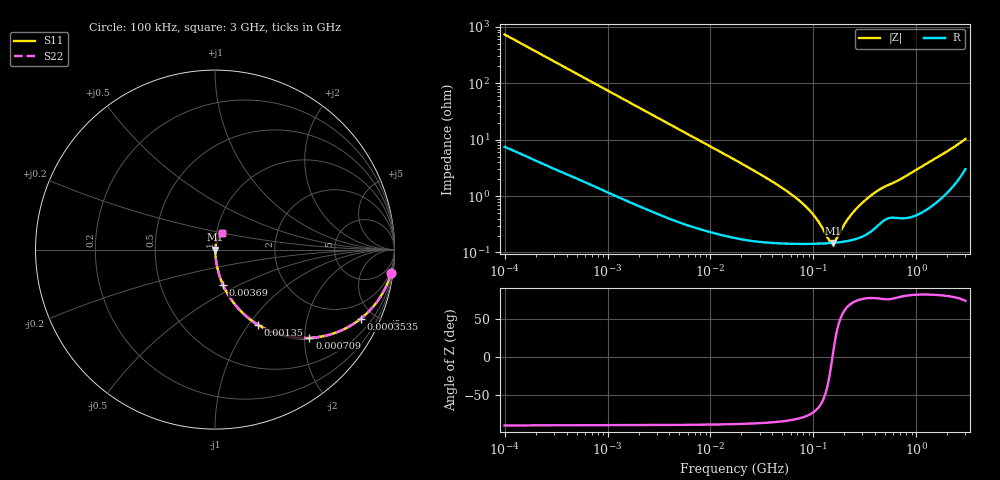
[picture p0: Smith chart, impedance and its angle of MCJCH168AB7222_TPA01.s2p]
! MCJCH168AB7222_TPA01  S-PARAMETER MODEL  ( Standard Model )
! Model Generated by TAIYO YUDEN Corporation (http://www.ty-top.com)
! Version 1.0
! TAIYO YUDEN Control No. 220601
! Copyright(c) 2015 TAIYO YUDEN CO.,LTD. All Rights Reserved.
! Product Description (link to TY-COMPAS)
! https://ds.yuden.co.jp/TYCOMPAS/or/detail?pn=MCJCH168AB7222KTPA01&u=M
! Products Name : Multilayer Ceramic Capacitors
! Characteristics :
!  Capacitance : 2200 [pF] , Rated Voltage : 100 [V] , TCC : X7R
!  Case Size : 1.6 x 0.8 / 0.063 x 0.031 [mm/inch] , Thickness : 0.8 / 0.031 [mm/inch]
!  (Conditions: Temperature = 25 [degC] , DC Bias Voltage = 0 [V])
! External Node Assignments :
!  1  o---| |---o  2
! GND o---------o GND
! Frequency Range : 100kHz  -  3GHz  [ 401 STEP ]
# MHZ S RI R 50
! Freq[MHz].  S11 Real  S11 Imag  S21 Real  S21 Imag  S12 Real  S12 Imag  S22 Real  S22 Imag
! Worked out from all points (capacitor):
!   401 points, 100 kHz to 3 GHz, reference 50 ohm
!   read as one part in series: C = 2.16 nF near 105.3 kHz
!   lowest |Z| = 148 mohm at 154.9 MHz (marker M1)
!   series resonance near 153.4 MHz, so ESL is about 500 pH
!   S11 on the Smith chart (normalised r, x): 100 kHz: 1, -15; 353.5 kHz: 1.05, -4.20; 709 kHz: 1.03, -2.11; 1.35 MHz: 1.02, -1.11; 3.69 MHz: 1.01, -0.41; 3 GHz: 1.06, +0.20
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0.1  0.9805 -0.1331  0.0195 0.1331  0.0195 0.1331  0.9805 -0.1331
0.205778  0.9256 -0.2568  0.0744 0.2568  0.0744 0.2568  0.9256 -0.2568
0.353547  0.812 -0.3844  0.188 0.3844  0.188 0.3844  0.812 -0.3844
0.562235  0.6354 -0.4743  0.3646 0.4743  0.3646 0.4743  0.6354 -0.4743
0.709011  0.5256 -0.492  0.4744 0.492  0.4744 0.492  0.5256 -0.492
1.350433  0.24 -0.4189  0.76 0.4189  0.76 0.4189  0.24 -0.4189
1.987766  0.1301 -0.3277  0.8699 0.3277  0.8699 0.3277  0.1301 -0.3277
3.161081  0.0582 -0.2245  0.9418 0.2245  0.9418 0.2245  0.0582 -0.2245
3.689712  0.0442 -0.1956  0.9558 0.1956  0.9558 0.1956  0.0442 -0.1956
7.399428  0.0131 -0.1013  0.9869 0.1013  0.9869 0.1013  0.0131 -0.1013
17.7727  0.00359 -0.0425  0.9964 0.0425  0.9964 0.0425  0.00359 -0.0425
53.83243  0.00159 -0.0126  0.9984 0.0126  0.9984 0.0126  0.00159 -0.0126
75.25761  0.00148 -0.00779  0.9985 0.00779  0.9985 0.00779  0.00148 -0.00779
97.38194  0.00144 -0.00474  0.9986 0.00474  0.9986 0.00474  0.00144 -0.00474
143.341  0.00146 -0.000687  0.9985 0.000687  0.9985 0.000687  0.00146 -0.000687
154.8634  0.00148 9.42e-05  0.9985 -9.42e-05  0.9985 -9.42e-05  0.00148 9.42e-05
167.3121  0.0015 0.000877  0.9985 -0.000877  0.9985 -0.000877  0.0015 0.000877
216.4987  0.00161 0.00357  0.9984 -0.00357  0.9984 -0.00357  0.00161 0.00357
273.0175  0.00182 0.00621  0.9982 -0.00621  0.9982 -0.00621  0.00182 0.00621
391.6425  0.00275 0.011  0.9973 -0.011  0.9973 -0.011  0.00275 0.011
547.5153  0.00431 0.0153  0.9957 -0.0153  0.9957 -0.0153  0.00431 0.0153
3000  0.0379 0.0918  0.9621 -0.0918  0.9621 -0.0918  0.0379 0.0918
